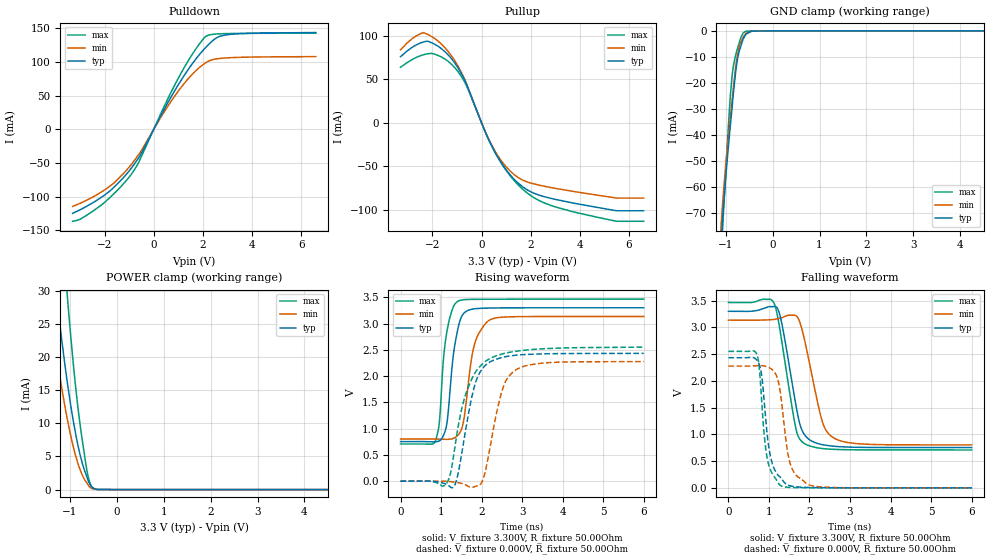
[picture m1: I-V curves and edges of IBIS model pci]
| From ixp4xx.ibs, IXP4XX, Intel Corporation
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[Model]   pci
Model_type   I/O
Vinl = 800.000mV
Vinh = 2.000V
Vmeas = 1.500V
Cref = 0.000F
|   typ   min   max
C_comp   3.000pF   2.700pF   3.300pF
[Voltage Range]   3.300V   3.135V   3.465V
[Temperature Range]   25.0   110.0   -40.0
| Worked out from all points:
|   slope of the pulldown table from 0 to 0.495 V, typ, clamps not added: 14.5 ohm
|   slope of the pullup table from 0 to 0.495 V, typ, clamps not added: 16 ohm
|   GND clamp passes 1 mA (typ) near -0.54 V on its own axis
|   POWER clamp passes 1 mA (typ) near -0.59 V on its own axis
|   falling waveform, V_fixture 3.300V, R_fixture 50.00Ohm: 20-80 % time 352ps typ, 398ps min, 346ps max; typ from 3.3 V to 0.753 V
|   rising waveform, V_fixture 3.300V, R_fixture 50.00Ohm: 20-80 % time 218ps typ, 269ps min, 187ps max; typ from 0.753 V to 3.3 V
|   rising waveform, V_fixture 0.000V, R_fixture 50.00Ohm: 20-80 % time 382ps typ, 386ps min, 507ps max; typ from 0 V to 2.43 V
|   falling waveform, V_fixture 0.000V, R_fixture 50.00Ohm: 20-80 % time 227ps typ, 250ps min, 186ps max; typ from 2.43 V to 0 V
[Pulldown]
|   Voltage   I(typ)   I(min)   I(max)
-3.3V     -124.6mA   -114.4mA   -136.4mA
-2.99V    -119.2mA   -109.6mA   -133.2mA
-1.99V    -97.22mA   -89.65mA   -108.2mA
-1.605V   -85.39mA   -79.22mA   -94.97mA
-885mV    -56.4mA    -50.94mA   -65.35mA
-525mV    -37.09mA   -32.82mA   -42.22mA
940mV     62.44mA    53.71mA    71.6mA
1.535V    95.49mA    80.32mA    109.3mA
2.08V     120mA      97.84mA    136.7mA
2.545V    135.5mA    104.5mA    141.4mA
2.89V     139.8mA    105.8mA    141.9mA
6.595V    143.5mA    107.9mA    142.6mA
[GND Clamp]
|   Voltage   I(typ)   I(min)   I(max)
-3.3V     -1.837A    -1.782A    -2.142A
-1.11V    -85.01mA   -78.04mA   -93.41mA
-1.065V   -72.56mA   -66.27mA   -76.24mA
-1.06V    -71.11mA   -65.16mA   -74.6mA
-925mV    -41.22mA   -37.4mA    -31.6mA
-860mV    -28.8mA    -26.04mA   -16.75mA
-790mV    -16.27mA   -14.37mA   -9.57mA
-750mV    -11.01mA   -9.296mA   -6.861mA
-675mV    -5.754mA   -4.387mA   -2.478mA
-580mV    -1.626mA   -1.201mA   -252.6uA
0V        -56.89nA   -17.57nA   -32.79pA
6.595V    0A         0A         0A
[Pullup]
|   Voltage   I(typ)   I(min)   I(max)
-3.3V     76.13mA    84.1mA     63.99mA
-2.365V   93.12mA    103.9mA    78.47mA
-1.77V    88.09mA    93.99mA    77.61mA
-1.165V   71.66mA    74.66mA    65.78mA
-670mV    48.06mA    48.83mA    45.84mA
475mV     -29.92mA   -28.79mA   -29.9mA
990mV     -53.5mA    -50.09mA   -54.15mA
1.545V    -70.51mA   -63.71mA   -72.8mA
2.15V     -81.02mA   -70.21mA   -86.2mA
3.05V     -88.15mA   -75.43mA   -96.88mA
5.5V      -100.9mA   -86.34mA   -113mA
6.595V    -100.9mA   -86.34mA   -113mA
[POWER Clamp]
|   Voltage   I(typ)   I(min)   I(max)
-3.3V     221.1mA    178.3mA    345.2mA
-1.5V     44.33mA    31.93mA    76.54mA
-1.44V    39.94mA    28.54mA    69.34mA
-1.27V    28.47mA    19.76mA    50.25mA
-1.06V    16.5mA     10.87mA    29.8mA
-1.045V   15.76mA    10.32mA    28.49mA
-890mV    8.924mA    5.478mA    16.42mA
-770mV    4.917mA    2.796mA    9.212mA
-635mV    1.89mA     986.7uA    2.845mA
-570mV    776uA      354.8uA    984.2uA
-515mV    310.8uA    129.8uA    274uA
6.595V    0A         0A         0A
[Ramp]
R_load = 50.00Ohm
|   typ   min   max
dV/dt_r   1.459V/380.412ps   1.366V/385.578ps   1.531V/506.912ps
dV/dt_f   1.528V/351.841ps   1.400V/398.136ps   1.654V/345.810ps
[Falling Waveform]
V_fixture = 3.300V
V_fixture_min = 3.135V
V_fixture_max = 3.465V
R_fixture = 50.00Ohm
|   Time   V(typ)   V(min)   V(max)
0s        3.3V       3.135V     3.465V
1.12ns    3.388V     3.148V     3.458V
1.21ns    3.354V     3.159V     3.215V
1.3ns     3.132V     3.177V     2.817V
1.66ns    1.569V     3.221V     1.126V
1.77ns    1.171V     3.077V     901.1mV
1.88ns    990.5mV    2.759V     825.8mV
2.3ns     810.2mV    1.281V     736.7mV
2.58ns    780mV      941.5mV    720.6mV
6ns       753.2mV    802.4mV    708.3mV
[Rising Waveform]
V_fixture = 3.300V
V_fixture_min = 3.135V
V_fixture_max = 3.465V
R_fixture = 50.00Ohm
|   Time   V(typ)   V(min)   V(max)
0s        753.2mV    802.4mV    708.3mV
860ps     748.4mV    801.8mV    762.9mV
960ps     769.3mV    799.7mV    1.133V
1.05ns    855.5mV    798.1mV    2.232V
1.13ns    1.039V     797mV      2.776V
1.41ns    2.877V     870.7mV    3.422V
1.56ns    3.194V     1.161V     3.454V
1.82ns    3.281V     2.589V     3.461V
2.19ns    3.295V     3.064V     3.463V
6ns       3.3V       3.135V     3.465V
[Rising Waveform]
V_fixture = 0.000V
V_fixture_min = 0.000V
V_fixture_max = 0.000V
R_fixture = 50.00Ohm
|   Time   V(typ)   V(min)   V(max)
0s        621.9nV    214.4nV    1.742nV
1.09ns    -46.28mV   -433.4uV   -78.62mV
1.32ns    -98.48mV   -15.59mV   537.4mV
1.53ns    618.2mV    -46.3mV    1.443V
1.84ns    1.849V     -101.2mV   2.065V
2.03ns    2.151V     20.24mV    2.238V
2.19ns    2.261V     563mV      2.328V
2.52ns    2.357V     1.757V     2.423V
2.85ns    2.398V     2.12V      2.473V
6ns       2.432V     2.276V     2.551V
[Falling Waveform]
V_fixture = 0.000V
V_fixture_min = 0.000V
V_fixture_max = 0.000V
R_fixture = 50.00Ohm
|   Time   V(typ)   V(min)   V(max)
0s        2.432V     2.276V     2.551V
700ps     2.389V     2.284V     2.498V
760ps     2.308V     2.285V     2.247V
820ps     2.097V     2.284V     1.626V
950ps     1.047V     2.264V     583.9mV
1.08ns    460.4mV    2.208V     267.8mV
1.3ns     182.7mV    1.671V     37.6mV
1.53ns    37mV       436mV      8.195mV
1.96ns    7.786mV    64.88mV    2.584mV
6ns       621.9nV    214.4nV    1.742nV
